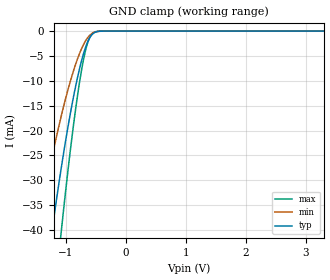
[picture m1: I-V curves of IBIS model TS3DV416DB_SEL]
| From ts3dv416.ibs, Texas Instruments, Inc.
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[Model]   TS3DV416DB_SEL
Model_type  Input
Vinl=0.8
Vinh=2.0
| variable   typ   min   max
C_comp   1.73pF   1.46pF   1.88pF
[Temperature Range]   40   100   -40
| Ambient temperature   25   85   -40
[Voltage range]   3.3   3   3.6
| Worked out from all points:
|   GND clamp passes 1 mA (typ) near -0.58 V on its own axis
[GND Clamp]
| TS3DV416DB_C
|   Voltage   I(typ)   I(min)   I(max)
-3.3V     -278.3mA   -199.9mA   -365.5mA
-1.475V   -63.03mA   -40.77mA   -90.95mA
-1.435V   -59.1mA    -38.09mA   -85.49mA
-1.23V    -40.17mA   -25.36mA   -58.72mA
-1.08V    -27.81mA   -17.26mA   -40.74mA
-1.065V   -26.66mA   -16.52mA   -39.03mA
-885mV    -14.03mA   -8.499mA   -20.12mA
-750mV    -6.535mA   -3.893mA   -8.727mA
-640mV    -2.291mA   -1.401mA   -2.516mA
-590mV    -1.125mA   -727.1uA   -1.027mA
-525mV    -332.6uA   -245.6uA   -218.1uA
3.3V      155.4pA    485pA      28.88pA
